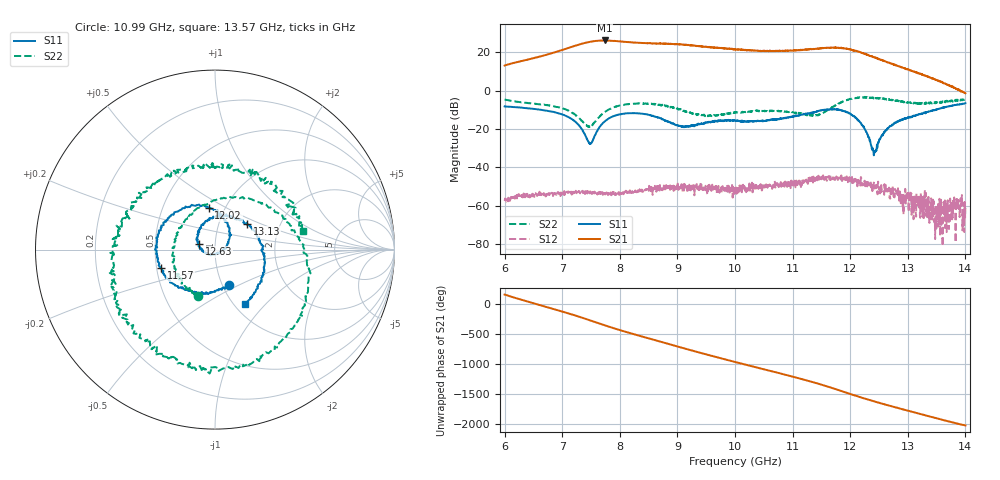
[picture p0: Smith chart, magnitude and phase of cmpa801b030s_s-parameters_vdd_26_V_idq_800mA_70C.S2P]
!Keysight Technologies,E5071C,MY46110325,B.14.03
!Date: Fri Aug 07 15:46:46 2020
!Data & Calibration Information:
!Freq	S11:SOLT2(ON)	S21:SOLT2(ON)	S12:SOLT2(ON)	S22:SOLT2(ON)
!PortZ  Port1:50+j0  Port2:50+j0
!Above PortZ is port z conversion or system Z0 setting when saving the data.
!When reading, reference impedance value at option line is always used.
# Hz S dB R 50
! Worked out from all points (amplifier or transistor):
!   1601 points, 6 GHz to 14 GHz, reference 50 ohm
!   highest |S21| = 26.2 dB at 7.74 GHz (marker M1)
!   |S21| within 3 dB of that: 7.199 GHz to 9.369 GHz (2.169 GHz wide, 26.2 % of centre)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
!   unconditionally stable (mu >= 1): start of sweep to end of sweep
!   at 7.33 GHz: K = 12.71, MAG = 24.5 dB, |S12| = -52.8 dB
!   at 10 GHz: K = 13.12, MAG = 22.0 dB, |S12| = -50.8 dB
!   at 14 GHz: K = 323.13, MAG = 1.8 dB, |S12| = -61.0 dB
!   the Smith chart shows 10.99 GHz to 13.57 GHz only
!   S11 on the Smith chart (normalised r, x): 10.99 GHz: 1.07, -0.44; 11.57 GHz: 0.53, -0.12; 12.02 GHz: 0.84, +0.41; 12.63 GHz: 0.84, +0.05; 13.13 GHz: 1.37, +0.41; 13.57 GHz: 1.12, -0.77
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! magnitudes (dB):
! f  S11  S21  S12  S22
! 6 GHz  -8.2  13.1  -57.4  -4.6
! 6.955 GHz  -11.9  20.8  -53.6  -8.8
! 7.335 GHz  -19.8  24.5  -53.0  -15.6
! 7.49 GHz  -27.8  25.5  -52.4  -18.6
! 7.74 GHz  -16.0  26.2  -53.5  -11.1
! 8.135 GHz  -11.7  25.4  -53.2  -7.0
! 8.67 GHz  -14.0  24.6  -48.9  -7.3
! 9.1 GHz  -18.6  23.9  -48.8  -10.5
! 10 GHz  -15.6  21.6  -50.8  -11.5
! 10.99 GHz  -13.6  20.8  -49.3  -11.1
! 11.34 GHz  -11.6  21.7  -46.6  -12.9
! 11.57 GHz  -9.9  22.3  -44.3  -10.7
! 12.02 GHz  -12.6  21.4  -46.8  -4.2
! 12.22 GHz  -18.4  19.6  -48.8  -3.6
! 12.41 GHz  -32.5  17.5  -49.8  -3.8
! 12.63 GHz  -20.5  15.0  -52.5  -4.7
! 12.67 GHz  -19.1  14.7  -52.5  -4.4
! 13.13 GHz  -12.7  9.7  -59.7  -6.6
! 13.57 GHz  -9.2  4.8  -63.0  -6.0
! 13.69 GHz  -8.3  3.1  -65.9  -5.5
! 13.78 GHz  -7.9  2.0  -59.7  -5.3
! 14 GHz  -6.5  -1.3  -61.0  -4.4
